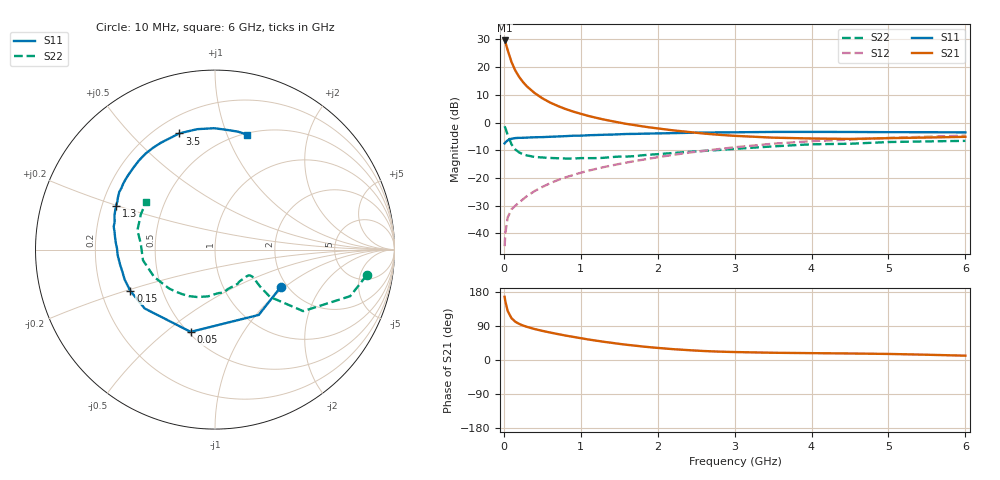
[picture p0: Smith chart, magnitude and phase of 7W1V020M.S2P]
! Infineon Technologies  Discrete & RF Semiconductors
! BFS17W
! Si NPN RF Bipolar Junction Transistor in SOT323
! VCE = 1 V  IC = 20 mA
! Common Emitter S-Parameters:  August  1999
# GHz  S  MA  R  50
!  f  S11  S21  S12  S22
! GHz  MAG  ANG  MAG  ANG  MAG  ANG  MAG  ANG
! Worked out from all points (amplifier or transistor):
!   36 points, 10 MHz to 6 GHz, reference 50 ohm
!   highest |S21| = 29.6 dB at 10 MHz (marker M1)
!   |S21| within 3 dB of that: start of sweep to 44.91 MHz
!   unconditionally stable (mu >= 1): 120 MHz to end of sweep
!   at 250 MHz: K = 1.48, MAG = 17.0 dB, |S12| = -27.7 dB
!   at 1.4 GHz: K = 1.64, MAG = 3.4 dB, |S12| = -15.5 dB
!   at 6 GHz: K = 1.14, MAG = -2.5 dB, |S12| = -4.7 dB
!   S11 on the Smith chart (normalised r, x): 10 MHz: 1.84, -0.94; 50 MHz: 0.51, -0.61; 150 MHz: 0.33, -0.21; 1.3 GHz: 0.26, +0.20; 3.5 GHz: 0.29, +0.70; 6 GHz: 0.51, +1.18
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0.01  0.421 -29.8  30.22 166.9  0.0059 76.5  0.8571 -9.6
0.02  0.4381 -56.2  28.18 154.5  0.0102 71.5  0.7968 -19.0
0.05  0.478 -106.5  20.22 129.3  0.0194 54.4  0.5992 -34.9
0.1  0.5111 -140.1  12.32 110.2  0.0273 49.7  0.4041 -40.7
0.15  0.5249 -154.0  8.615 100.9  0.0317 50.8  0.3256 -39.4
0.2  0.5304 -161.7  6.621 95.2  0.0363 54.7  0.2889 -37.6
0.25  0.5309 -167.1  5.35 90.9  0.0414 56.7  0.2676 -36.1
0.3  0.5352 -170.8  4.487 87.5  0.0472 59.2  0.2553 -35.9
0.4  0.5431 -176.7  3.408 81.7  0.0581 62.3  0.2398 -36.6
0.5  0.5461 179.3  2.742 76.9  0.069 64.7  0.2345 -38.2
0.6  0.5539 176.1  2.3 72.6  0.0804 65.9  0.2299 -40.9
0.7  0.561 173.0  1.993 68.5  0.0916 66.5  0.2273 -44.7
0.9  0.5785 167.3  1.579 61.1  0.1131 66.9  0.2241 -53.0
1.1  0.5907 161.5  1.316 54.1  0.1355 66.7  0.2281 -62.1
1.3  0.6023 156.1  1.133 48.0  0.1574 66.0  0.2312 -71.9
1.6  0.6227 148.9  0.943 40.1  0.1904 64.9  0.2433 -85.6
2.2  0.6442 134.8  0.723 28.6  0.2612 61.3  0.2826 -110.9
2.8  0.6641 121.2  0.601 22.1  0.3332 55.4  0.3207 -133.3
3.5  0.6773 107.1  0.534 19.1  0.4153 47.0  0.3716 -155.7
4.5  0.6764 90.5  0.507 17.2  0.4925 34.1  0.4146 175.6
5.5  0.6695 79.0  0.537 13.9  0.5546 23.7  0.4573 154.6
6  0.6653 74.4  0.553 11.4  0.5817 18.7  0.4675 145.1
